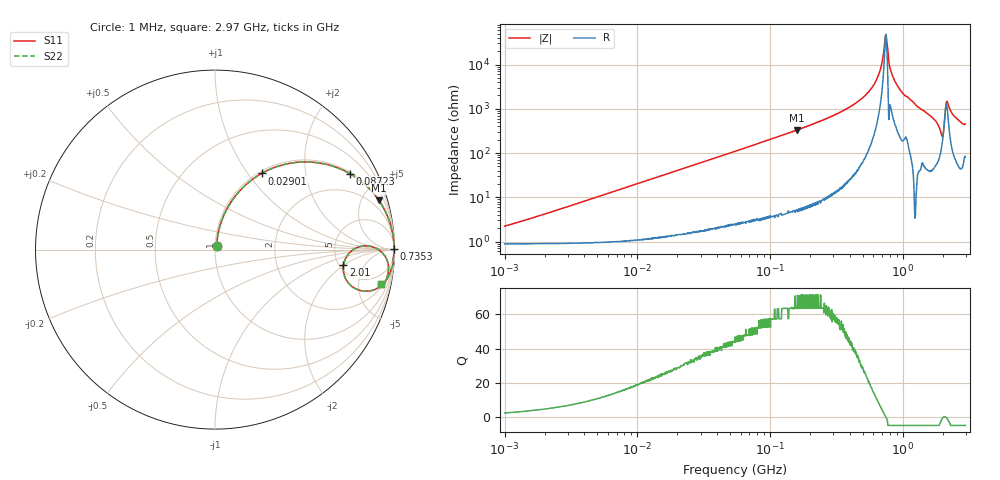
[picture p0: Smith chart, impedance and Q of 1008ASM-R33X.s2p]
!s-Parameter Generated by FASTRON Sdn. Bhd.
!FASTRON P/N : 1008ASM-R33X
!Keysight Technologies: E4991B_MY54100416_A.01.15
!Date: Tue Nov 21 09:10:56 2023
!Version  :Rev00  Wed Nov 22 15:14:33 2023
!Data & Calibration Information:
!Freq  S11  S21  S12  S22
!PortZ  Port1:50+j0  Port2:50+j0
!When reading reference impedance value at option line is always used.
! Remarks : This data is being provided solely for informational purposes.
# Hz S dB R 50
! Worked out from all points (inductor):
!   1599 points, 1 MHz to 2.97 GHz, reference 50 ohm
!   read as one part in series: L = 325 nH near 1.31 MHz
!   highest Q = 63.9 at 159 MHz (marker M1), where L = 331 nH
!   self-resonance near 742.7 MHz
!   S11 on the Smith chart (normalised r, x): 1 MHz: 1.02, +0.04; 29.01 MHz: 1.03, +1.17; 87.23 MHz: 1.07, +3.51; 735.3 MHz: open; 2.01 GHz: 5.43, -1.95; 2.97 GHz: 2.65, -8.99
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1000000  -33.10 65.4  -0.08 -1.2  -0.08 -1.2  -33.10 65.4
3804036  -22.30 78.8  -0.11 -4.4  -0.11 -4.4  -22.30 78.8
1.439846e7  -11.20 71.5  -0.45 -16.0  -0.45 -16.0  -11.20 71.5
2.90111e7  -6.06 58.5  -1.38 -29.8  -1.38 -29.8  -6.06 58.5
5.477226e7  -2.72 41.7  -3.53 -47.0  -3.53 -47.0  -2.72 41.7
8.723049e7  -1.29 29.4  -6.18 -59.5  -6.18 -59.5  -1.29 29.4
1.590202e8  -0.42 16.8  -10.80 -72.3  -10.80 -72.3  -0.42 16.8
2.073156e8  -0.24 12.7  -13.20 -76.5  -13.20 -76.5  -0.24 12.7
3.798301e8  -0.06 5.7  -20.10 -83.1  -20.10 -83.1  -0.06 5.7
5.418594e8  -0.03 2.5  -27.10 -84.9  -27.10 -84.9  -0.03 2.5
6.586299e8  -0.02 1.0  -35.40 -82.0  -35.40 -82.0  -0.02 1.0
7.352784e8  -0.02 0.1  -50.90 -41.7  -50.90 -41.7  -0.02 0.1
7.576891e8  -0.02 -0.1  -51.20 44.2  -51.20 44.2  -0.02 -0.1
7.846996e8  -0.00 -0.5  -41.80 86.6  -41.80 86.6  -0.00 -0.5
8.416437e8  -0.02 -1.0  -34.70 81.9  -34.70 81.9  -0.02 -1.0
9.878038e8  -0.04 -2.4  -27.50 83.0  -27.50 83.0  -0.04 -2.4
1.721456e9  -0.24 -9.6  -15.50 75.9  -15.50 75.9  -0.24 -9.6
1.912199e9  -0.93 -14.8  -11.60 60.1  -11.60 60.1  -0.93 -14.8
2.01032e9  -2.85 -6.9  -10.50 16.9  -10.50 16.9  -2.85 -6.9
2.177892e9  -0.38 -3.1  -23.30 49.4  -23.30 49.4  -0.38 -3.1
2.455801e9  -0.24 -8.2  -16.80 75.0  -16.80 75.0  -0.24 -8.2
2.970126e9  -0.52 -11.7  -13.70 67.9  -13.70 67.9  -0.52 -11.7
